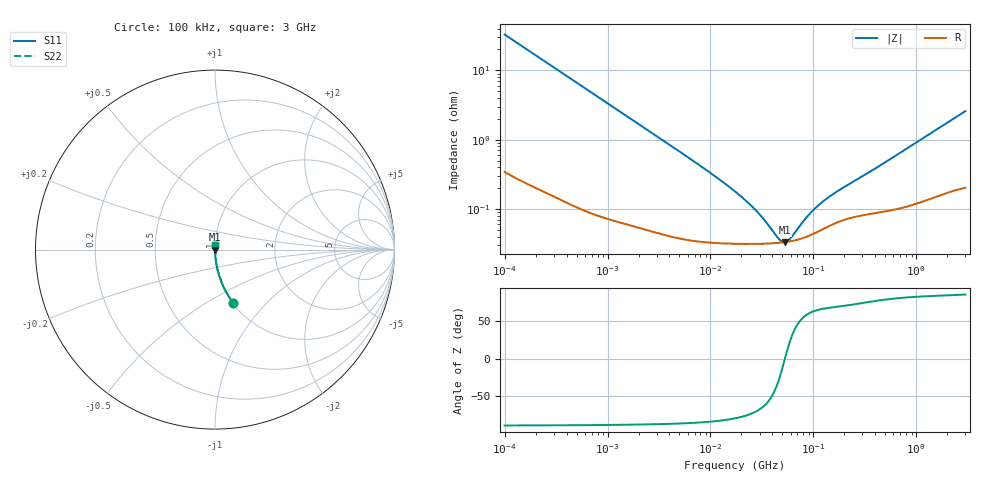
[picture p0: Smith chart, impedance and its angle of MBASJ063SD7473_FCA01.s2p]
! MBASJ063SD7473_FCA01  S-PARAMETER MODEL  ( Standard Model )
! Model Generated by TAIYO YUDEN Corporation (http://www.ty-top.com)
! Version 1.0
! TAIYO YUDEN Control No. 220601
! Copyright(c) 2022 TAIYO YUDEN CO.,LTD. All Rights Reserved.
! Product Description (link to TY-COMPAS)
! https://ds.yuden.co.jp/TYCOMPAS/or/detail?pn=MBASJ063SD7473KFCA01&u=M
! Products Name : Multilayer Ceramic Capacitors
! Characteristics :
!  Capacitance : 0.047 [uF] , Rated Voltage : 6.3 [V] , TCC : X7T
!  Case Size : 0.6 x 0.3 / 0.024 x 0.012 [mm/inch] , Thickness : 0.3 / 0.012 [mm/inch]
!  (Conditions: Temperature = 25 [degC] , DC Bias Voltage = 0 [V])
! External Node Assignments :
!  1  o---| |---o  2
! GND o---------o GND
! Frequency Range : 100kHz  -  3GHz  [ 401 STEP ]
# MHZ S RI R 50
! Freq[MHz].  S11 Real  S11 Imag  S21 Real  S21 Imag  S12 Real  S12 Imag  S22 Real  S22 Imag
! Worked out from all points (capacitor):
!   401 points, 100 kHz to 3 GHz, reference 50 ohm
!   read as one part in series: C = 48.2 nF near 105.3 kHz
!   lowest |Z| = 33.2 mohm at 52.46 MHz (marker M1)
!   series resonance near 52.96 MHz, so ESL is about 190 pH
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0.1  0.1004 -0.2953  0.8996 0.2953  0.8996 0.2953  0.1004 -0.2953
0.147195  0.05 -0.2125  0.95 0.2125  0.95 0.2125  0.05 -0.2125
0.228123  0.0223 -0.1416  0.9777 0.1416  0.9777 0.1416  0.0223 -0.1416
0.562235  0.00447 -0.0589  0.9955 0.0589  0.9955 0.0589  0.00447 -0.0589
1.18716  0.00146 -0.0281  0.9985 0.0281  0.9985 0.0281  0.00146 -0.0281
3.161081  0.000556 -0.0107  0.9994 0.0107  0.9994 0.0107  0.000556 -0.0107
9.331111  0.000341 -0.00354  0.9997 0.00354  0.9997 0.00354  0.000341 -0.00354
17.7727  0.000317 -0.00171  0.9997 0.00171  0.9997 0.00171  0.000317 -0.00171
22.99754  0.000314 -0.00121  0.9997 0.00121  0.9997 0.00121  0.000314 -0.00121
29.00125  0.000315 -0.000827  0.9997 0.000827  0.9997 0.000827  0.000315 -0.000827
33.85116  0.000316 -0.000599  0.9997 0.000599  0.9997 0.000599  0.000316 -0.000599
46.11977  0.000325 -0.00018  0.9997 0.00018  0.9997 0.00018  0.000325 -0.00018
49.82709  0.000328 -7.92e-05  0.9997 7.92e-05  0.9997 7.92e-05  0.000328 -7.92e-05
52.46276  0.000332 -1.22e-05  0.9997 1.22e-05  0.9997 1.22e-05  0.000332 -1.22e-05
55.23785  0.000335 5.47e-05  0.9997 -5.47e-05  0.9997 -5.47e-05  0.000335 5.47e-05
59.67813  0.000342 0.000155  0.9997 -0.000155  0.9997 -0.000155  0.000342 0.000155
81.30716  0.000386 0.000569  0.9996 -0.000569  0.9996 -0.000569  0.000386 0.000569
97.38194  0.00043 0.000823  0.9996 -0.000823  0.9996 -0.000823  0.00043 0.000823
122.8043  0.000509 0.00116  0.9995 -0.00116  0.9995 -0.00116  0.000509 0.00116
158.9065  0.000613 0.00156  0.9994 -0.00156  0.9994 -0.00156  0.000613 0.00156
547.5153  0.00097 0.00505  0.999 -0.00505  0.999 -0.00505  0.00097 0.00505
3000  0.00268 0.0256  0.9973 -0.0256  0.9973 -0.0256  0.00268 0.0256
